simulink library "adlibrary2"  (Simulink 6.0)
settings: Solver=ode45  StartTime=0.0  StopTime=10.0  RelTol=1e-3
undefined symbols (not defined in the file or in its folder): adlibrary2, ADM, Bit, DDR, Generation, II, Location, Lower, SDRAM, SRAM, Width, XP, XPL, XRC, ZBT
libraries: xbsIndex_r3 x581, adlibrary2 x2
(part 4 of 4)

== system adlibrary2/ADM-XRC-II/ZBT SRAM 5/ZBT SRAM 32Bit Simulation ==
  d : Inport  Port=1  LatchInput=off
  a : Inport  Port=2  LatchInput=off
  w : Inport  Port=3  LatchInput=off
  r : Inport  Port=4  LatchInput=off
  be : Inport  Port=5  LatchInput=off
  Disregard Subsystem : xbsIndex_r3/Disregard Subsystem  Tag=discardX
  Gateway In6 : xbsIndex_r3/Gateway In  arith_type=Boolean  n_bits=1  bin_pt=0  quantization=Truncate  overflow=Wrap  period=1  timing_constraint=None  locs_specified=off  LOCs={}  needs_fixed_name=off  dbl_ovrd=on  show_param=off
  Gateway In7 : xbsIndex_r3/Gateway In  arith_type=Unsigned  n_bits=32  bin_pt=0  quantization=Truncate  overflow=Wrap  period=1  timing_constraint=None  locs_specified=off  LOCs={}  needs_fixed_name=off  dbl_ovrd=on  show_param=off
  Gateway Out{,1..4} (5 alike) : xbsIndex_r3/Gateway Out  hdl_port=off  timing_constraint=None  locs_specified=off  LOCs={}  needs_fixed_name=off  show_param=off
  S-Function : S-Function  FunctionName=zbt32
  q : Outport
  qv : Outport  Port=2
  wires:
  S-Function/2 -> Gateway In6/1
  Gateway In7/1 -> q/1
  Gateway In6/1 -> qv/1
  Gateway Out3/1 -> S-Function/4
  Gateway Out2/1 -> S-Function/3
  Gateway Out1/1 -> S-Function/2
  Gateway Out/1 -> S-Function/1
  S-Function/1 -> Gateway In7/1
  r/1 -> Gateway Out3/1
  w/1 -> Gateway Out2/1
  a/1 -> Gateway Out1/1
  d/1 -> Gateway Out/1
  Gateway Out4/1 -> S-Function/5
  be/1 -> Gateway Out4/1

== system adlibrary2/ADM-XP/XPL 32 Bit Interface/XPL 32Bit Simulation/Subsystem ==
  In1 : Inport  Port=1  LatchInput=off
  In2 : Inport  Port=2  LatchInput=off
  In9 : Inport  Port=3  LatchInput=off
  In3 : Inport  Port=4  LatchInput=off
  In4 : Inport  Port=5  LatchInput=off
  In5 : Inport  Port=6  LatchInput=off
  In6 : Inport  Port=7  LatchInput=off
  In7 : Inport  Port=8  LatchInput=off
  In8 : Inport  Port=9  LatchInput=off
  Disregard Subsystem : xbsIndex_r3/Disregard Subsystem  Tag=discardX
  Gateway In{,1,4..5} (4 alike) : xbsIndex_r3/Gateway In  arith_type=Boolean  n_bits=8  bin_pt=6  quantization=Truncate  overflow=Wrap  period=1  timing_constraint=None  locs_specified=off  LOCs={}  needs_fixed_name=off  dbl_ovrd=off  show_param=off
  Gateway In2 : xbsIndex_r3/Gateway In  arith_type=Unsigned  n_bits=32  bin_pt=0  quantization=Truncate  overflow=Wrap  period=1  timing_constraint=None  locs_specified=off  LOCs={}  needs_fixed_name=off  dbl_ovrd=off  show_param=off
  Gateway In3 : xbsIndex_r3/Gateway In  arith_type=Unsigned  n_bits=32  bin_pt=0  quantization=Truncate  overflow=Wrap  period=1  timing_constraint=None  locs_specified=off  LOCs={}  needs_fixed_name=off  dbl_ovrd=off  show_param=off
  Gateway In6 : xbsIndex_r3/Gateway In  arith_type=Unsigned  n_bits=16  bin_pt=0  quantization=Truncate  overflow=Wrap  period=1  timing_constraint=None  locs_specified=off  LOCs={}  needs_fixed_name=off  dbl_ovrd=off  show_param=off
  Gateway In7 : xbsIndex_r3/Gateway In  arith_type=Unsigned  n_bits=32  bin_pt=0  quantization=Truncate  overflow=Wrap  period=1  timing_constraint=None  locs_specified=off  LOCs={}  needs_fixed_name=off  dbl_ovrd=off  show_param=off
  Gateway In8 : xbsIndex_r3/Gateway In  arith_type=Unsigned  n_bits=4  bin_pt=0  quantization=Truncate  overflow=Wrap  period=1  timing_constraint=None  locs_specified=off  LOCs={}  needs_fixed_name=off  dbl_ovrd=off  show_param=off
  Out1 : Outport
  Out2 : Outport  Port=2
  Out9 : Outport  Port=3
  Out3 : Outport  Port=4
  Out4 : Outport  Port=5
  Out5 : Outport  Port=6
  Out6 : Outport  Port=7
  Out7 : Outport  Port=8
  Out8 : Outport  Port=9
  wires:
  In1/1 -> Gateway In7/1
  In2/1 -> Gateway In6/1
  In3/1 -> Gateway In5/1
  In4/1 -> Gateway In4/1
  In5/1 -> Gateway In3/1
  In6/1 -> Gateway In2/1
  In7/1 -> Gateway In1/1
  In8/1 -> Gateway In/1
  Gateway In/1 -> Out8/1
  Gateway In1/1 -> Out7/1
  Gateway In2/1 -> Out6/1
  Gateway In3/1 -> Out5/1
  Gateway In4/1 -> Out4/1
  Gateway In5/1 -> Out3/1
  Gateway In6/1 -> Out2/1
  Gateway In7/1 -> Out1/1
  In9/1 -> Gateway In8/1
  Gateway In8/1 -> Out9/1

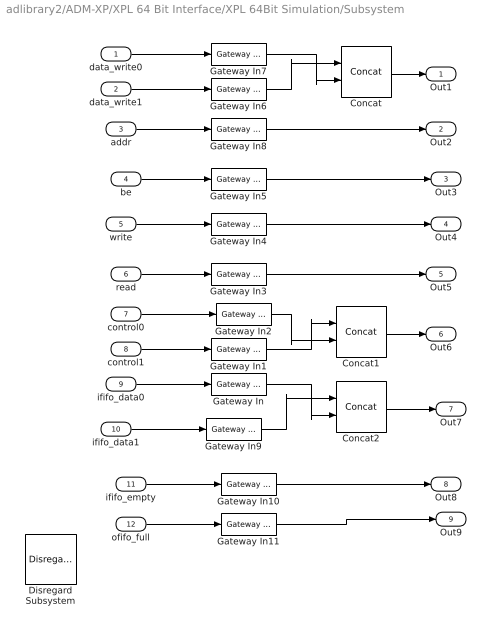
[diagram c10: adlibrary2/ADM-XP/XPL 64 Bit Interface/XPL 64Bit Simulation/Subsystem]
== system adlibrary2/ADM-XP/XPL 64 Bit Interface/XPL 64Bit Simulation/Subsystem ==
  data_write0 : Inport  Port=1  LatchInput=off
  data_write1 : Inport  Port=2  LatchInput=off
  addr : Inport  Port=3  LatchInput=off
  be : Inport  Port=4  LatchInput=off
  write : Inport  Port=5  LatchInput=off
  read : Inport  Port=6  LatchInput=off
  control0 : Inport  Port=7  LatchInput=off
  control1 : Inport  Port=8  LatchInput=off
  ififo_data0 : Inport  Port=9  LatchInput=off
  ififo_data1 : Inport  Port=10  LatchInput=off
  ififo_empty : Inport  Port=11  LatchInput=off
  ofifo_full : Inport  Port=12  LatchInput=off
  Concat : xbsIndex_r3/Concat  num_inputs=2  explicit_period=off  period=1  dbl_ovrd=off
  Concat1 : xbsIndex_r3/Concat  num_inputs=2  explicit_period=off  period=1  dbl_ovrd=off
  Concat2 : xbsIndex_r3/Concat  num_inputs=2  explicit_period=off  period=1  dbl_ovrd=off
  Disregard Subsystem : xbsIndex_r3/Disregard Subsystem  Tag=discardX
  Gateway In{,1..2,6..7,9} (6 alike) : xbsIndex_r3/Gateway In  arith_type=Unsigned  n_bits=32  bin_pt=0  quantization=Truncate  overflow=Wrap  period=1  timing_constraint=None  locs_specified=off  LOCs={}  needs_fixed_name=off  dbl_ovrd=off  show_param=off
  Gateway In10 : xbsIndex_r3/Gateway In  arith_type=Boolean  n_bits=8  bin_pt=6  quantization=Truncate  overflow=Wrap  period=1  timing_constraint=None  locs_specified=off  LOCs={}  needs_fixed_name=off  dbl_ovrd=off  show_param=off
  Gateway In11 : xbsIndex_r3/Gateway In  arith_type=Boolean  n_bits=8  bin_pt=6  quantization=Truncate  overflow=Wrap  period=1  timing_constraint=None  locs_specified=off  LOCs={}  needs_fixed_name=off  dbl_ovrd=off  show_param=off
  Gateway In3 : xbsIndex_r3/Gateway In  arith_type=Boolean  n_bits=32  bin_pt=0  quantization=Truncate  overflow=Wrap  period=1  timing_constraint=None  locs_specified=off  LOCs={}  needs_fixed_name=off  dbl_ovrd=off  show_param=off
  Gateway In4 : xbsIndex_r3/Gateway In  arith_type=Boolean  n_bits=8  bin_pt=6  quantization=Truncate  overflow=Wrap  period=1  timing_constraint=None  locs_specified=off  LOCs={}  needs_fixed_name=off  dbl_ovrd=off  show_param=off
  Gateway In5 : xbsIndex_r3/Gateway In  arith_type=Unsigned  n_bits=8  bin_pt=0  quantization=Truncate  overflow=Wrap  period=1  timing_constraint=None  locs_specified=off  LOCs={}  needs_fixed_name=off  dbl_ovrd=off  show_param=off
  Gateway In8 : xbsIndex_r3/Gateway In  arith_type=Unsigned  n_bits=16  bin_pt=0  quantization=Truncate  overflow=Wrap  period=1  timing_constraint=None  locs_specified=off  LOCs={}  needs_fixed_name=off  dbl_ovrd=off  show_param=off
  Out1 : Outport
  Out2 : Outport  Port=2
  Out3 : Outport  Port=3
  Out4 : Outport  Port=4
  Out5 : Outport  Port=5
  Out6 : Outport  Port=6
  Out7 : Outport  Port=7
  Out8 : Outport  Port=8
  Out9 : Outport  Port=9
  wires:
  Gateway In11/1 -> Out9/1
  Gateway In10/1 -> Out8/1
  Concat2/1 -> Out7/1
  Gateway In/1 -> Concat2/2
  Gateway In9/1 -> Concat2/1
  ofifo_full/1 -> Gateway In11/1
  ififo_empty/1 -> Gateway In10/1
  ififo_data1/1 -> Gateway In9/1
  Concat1/1 -> Out6/1
  Gateway In1/1 -> Concat1/1
  Gateway In2/1 -> Concat1/2
  Gateway In3/1 -> Out5/1
  Gateway In4/1 -> Out4/1
  Gateway In5/1 -> Out3/1
  Gateway In8/1 -> Out2/1
  Concat/1 -> Out1/1
  Gateway In7/1 -> Concat/2
  Gateway In6/1 -> Concat/1
  addr/1 -> Gateway In8/1
  ififo_data0/1 -> Gateway In/1
  control1/1 -> Gateway In1/1
  control0/1 -> Gateway In2/1
  read/1 -> Gateway In3/1
  write/1 -> Gateway In4/1
  be/1 -> Gateway In5/1
  data_write1/1 -> Gateway In6/1
  data_write0/1 -> Gateway In7/1

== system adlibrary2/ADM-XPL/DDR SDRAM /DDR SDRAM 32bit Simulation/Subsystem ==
  In1 : Inport  Port=1  LatchInput=off
  In2 : Inport  Port=2  LatchInput=off
  In3 : Inport  Port=3  LatchInput=off
  Disregard Subsystem : xbsIndex_r3/Disregard Subsystem  Tag=discardX
  g02 : xbsIndex_r3/Gateway In  arith_type=Unsigned  n_bits=3  bin_pt=0  quantization=Truncate  overflow=Wrap  period=1  timing_constraint=None  locs_specified=off  LOCs={}  needs_fixed_name=off  dbl_ovrd=off  show_param=off
  go0 : xbsIndex_r3/Gateway In  arith_type=Unsigned  n_bits=32  bin_pt=0  quantization=Truncate  overflow=Wrap  period=1  timing_constraint=None  locs_specified=off  LOCs={}  needs_fixed_name=off  dbl_ovrd=off  show_param=off
  go1 : xbsIndex_r3/Gateway In  arith_type=Boolean  n_bits=32  bin_pt=0  quantization=Truncate  overflow=Wrap  period=1  timing_constraint=None  locs_specified=off  LOCs={}  needs_fixed_name=off  dbl_ovrd=off  show_param=off
  Out1 : Outport
  Out2 : Outport  Port=2
  Out3 : Outport  Port=3
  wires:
  In1/1 -> go0/1
  In2/1 -> go1/1
  In3/1 -> g02/1
  go0/1 -> Out1/1
  go1/1 -> Out2/1
  g02/1 -> Out3/1

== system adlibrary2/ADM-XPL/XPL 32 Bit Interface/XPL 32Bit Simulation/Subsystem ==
  In1 : Inport  Port=1  LatchInput=off
  In2 : Inport  Port=2  LatchInput=off
  In9 : Inport  Port=3  LatchInput=off
  In3 : Inport  Port=4  LatchInput=off
  In4 : Inport  Port=5  LatchInput=off
  In5 : Inport  Port=6  LatchInput=off
  In6 : Inport  Port=7  LatchInput=off
  In7 : Inport  Port=8  LatchInput=off
  In8 : Inport  Port=9  LatchInput=off
  Disregard Subsystem : xbsIndex_r3/Disregard Subsystem  Tag=discardX
  Gateway In{,1,4..5} (4 alike) : xbsIndex_r3/Gateway In  arith_type=Boolean  n_bits=8  bin_pt=6  quantization=Truncate  overflow=Wrap  period=1  timing_constraint=None  locs_specified=off  LOCs={}  needs_fixed_name=off  dbl_ovrd=off  show_param=off
  Gateway In2 : xbsIndex_r3/Gateway In  arith_type=Unsigned  n_bits=32  bin_pt=0  quantization=Truncate  overflow=Wrap  period=1  timing_constraint=None  locs_specified=off  LOCs={}  needs_fixed_name=off  dbl_ovrd=off  show_param=off
  Gateway In3 : xbsIndex_r3/Gateway In  arith_type=Unsigned  n_bits=32  bin_pt=0  quantization=Truncate  overflow=Wrap  period=1  timing_constraint=None  locs_specified=off  LOCs={}  needs_fixed_name=off  dbl_ovrd=off  show_param=off
  Gateway In6 : xbsIndex_r3/Gateway In  arith_type=Unsigned  n_bits=16  bin_pt=0  quantization=Truncate  overflow=Wrap  period=1  timing_constraint=None  locs_specified=off  LOCs={}  needs_fixed_name=off  dbl_ovrd=off  show_param=off
  Gateway In7 : xbsIndex_r3/Gateway In  arith_type=Unsigned  n_bits=32  bin_pt=0  quantization=Truncate  overflow=Wrap  period=1  timing_constraint=None  locs_specified=off  LOCs={}  needs_fixed_name=off  dbl_ovrd=off  show_param=off
  Gateway In8 : xbsIndex_r3/Gateway In  arith_type=Unsigned  n_bits=4  bin_pt=0  quantization=Truncate  overflow=Wrap  period=1  timing_constraint=None  locs_specified=off  LOCs={}  needs_fixed_name=off  dbl_ovrd=off  show_param=off
  Out1 : Outport
  Out2 : Outport  Port=2
  Out9 : Outport  Port=3
  Out3 : Outport  Port=4
  Out4 : Outport  Port=5
  Out5 : Outport  Port=6
  Out6 : Outport  Port=7
  Out7 : Outport  Port=8
  Out8 : Outport  Port=9
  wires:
  Gateway In8/1 -> Out9/1
  In9/1 -> Gateway In8/1
  Gateway In7/1 -> Out1/1
  Gateway In6/1 -> Out2/1
  Gateway In5/1 -> Out3/1
  Gateway In4/1 -> Out4/1
  Gateway In3/1 -> Out5/1
  Gateway In2/1 -> Out6/1
  Gateway In1/1 -> Out7/1
  Gateway In/1 -> Out8/1
  In8/1 -> Gateway In/1
  In7/1 -> Gateway In1/1
  In6/1 -> Gateway In2/1
  In5/1 -> Gateway In3/1
  In4/1 -> Gateway In4/1
  In3/1 -> Gateway In5/1
  In2/1 -> Gateway In6/1
  In1/1 -> Gateway In7/1

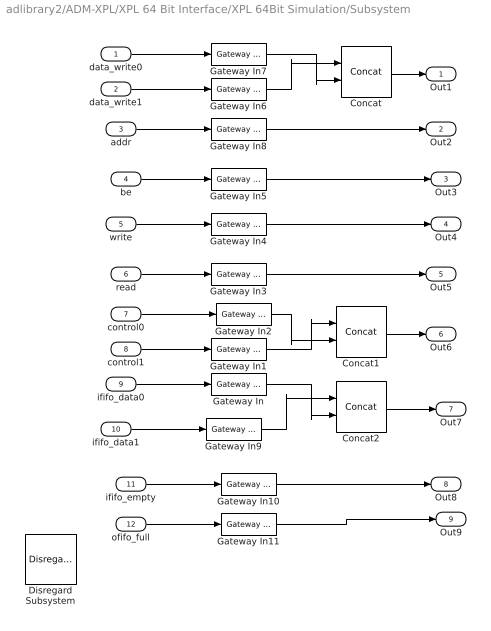
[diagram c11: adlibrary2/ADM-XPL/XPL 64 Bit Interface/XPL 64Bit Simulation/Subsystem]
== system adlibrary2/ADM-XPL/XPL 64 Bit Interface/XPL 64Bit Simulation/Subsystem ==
  data_write0 : Inport  Port=1  LatchInput=off
  data_write1 : Inport  Port=2  LatchInput=off
  addr : Inport  Port=3  LatchInput=off
  be : Inport  Port=4  LatchInput=off
  write : Inport  Port=5  LatchInput=off
  read : Inport  Port=6  LatchInput=off
  control0 : Inport  Port=7  LatchInput=off
  control1 : Inport  Port=8  LatchInput=off
  ififo_data0 : Inport  Port=9  LatchInput=off
  ififo_data1 : Inport  Port=10  LatchInput=off
  ififo_empty : Inport  Port=11  LatchInput=off
  ofifo_full : Inport  Port=12  LatchInput=off
  Concat : xbsIndex_r3/Concat  num_inputs=2  explicit_period=off  period=1  dbl_ovrd=off
  Concat1 : xbsIndex_r3/Concat  num_inputs=2  explicit_period=off  period=1  dbl_ovrd=off
  Concat2 : xbsIndex_r3/Concat  num_inputs=2  explicit_period=off  period=1  dbl_ovrd=off
  Disregard Subsystem : xbsIndex_r3/Disregard Subsystem  Tag=discardX
  Gateway In{,1..2,6..7,9} (6 alike) : xbsIndex_r3/Gateway In  arith_type=Unsigned  n_bits=32  bin_pt=0  quantization=Truncate  overflow=Wrap  period=1  timing_constraint=None  locs_specified=off  LOCs={}  needs_fixed_name=off  dbl_ovrd=off  show_param=off
  Gateway In10 : xbsIndex_r3/Gateway In  arith_type=Boolean  n_bits=8  bin_pt=6  quantization=Truncate  overflow=Wrap  period=1  timing_constraint=None  locs_specified=off  LOCs={}  needs_fixed_name=off  dbl_ovrd=off  show_param=off
  Gateway In11 : xbsIndex_r3/Gateway In  arith_type=Boolean  n_bits=8  bin_pt=6  quantization=Truncate  overflow=Wrap  period=1  timing_constraint=None  locs_specified=off  LOCs={}  needs_fixed_name=off  dbl_ovrd=off  show_param=off
  Gateway In3 : xbsIndex_r3/Gateway In  arith_type=Boolean  n_bits=32  bin_pt=0  quantization=Truncate  overflow=Wrap  period=1  timing_constraint=None  locs_specified=off  LOCs={}  needs_fixed_name=off  dbl_ovrd=off  show_param=off
  Gateway In4 : xbsIndex_r3/Gateway In  arith_type=Boolean  n_bits=8  bin_pt=6  quantization=Truncate  overflow=Wrap  period=1  timing_constraint=None  locs_specified=off  LOCs={}  needs_fixed_name=off  dbl_ovrd=off  show_param=off
  Gateway In5 : xbsIndex_r3/Gateway In  arith_type=Unsigned  n_bits=8  bin_pt=0  quantization=Truncate  overflow=Wrap  period=1  timing_constraint=None  locs_specified=off  LOCs={}  needs_fixed_name=off  dbl_ovrd=off  show_param=off
  Gateway In8 : xbsIndex_r3/Gateway In  arith_type=Unsigned  n_bits=16  bin_pt=0  quantization=Truncate  overflow=Wrap  period=1  timing_constraint=None  locs_specified=off  LOCs={}  needs_fixed_name=off  dbl_ovrd=off  show_param=off
  Out1 : Outport
  Out2 : Outport  Port=2
  Out3 : Outport  Port=3
  Out4 : Outport  Port=4
  Out5 : Outport  Port=5
  Out6 : Outport  Port=6
  Out7 : Outport  Port=7
  Out8 : Outport  Port=8
  Out9 : Outport  Port=9
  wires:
  data_write0/1 -> Gateway In7/1
  data_write1/1 -> Gateway In6/1
  be/1 -> Gateway In5/1
  write/1 -> Gateway In4/1
  read/1 -> Gateway In3/1
  control0/1 -> Gateway In2/1
  control1/1 -> Gateway In1/1
  ififo_data0/1 -> Gateway In/1
  addr/1 -> Gateway In8/1
  Gateway In6/1 -> Concat/1
  Gateway In7/1 -> Concat/2
  Concat/1 -> Out1/1
  Gateway In8/1 -> Out2/1
  Gateway In5/1 -> Out3/1
  Gateway In4/1 -> Out4/1
  Gateway In3/1 -> Out5/1
  Gateway In2/1 -> Concat1/2
  Gateway In1/1 -> Concat1/1
  Concat1/1 -> Out6/1
  ififo_data1/1 -> Gateway In9/1
  ififo_empty/1 -> Gateway In10/1
  ofifo_full/1 -> Gateway In11/1
  Gateway In9/1 -> Concat2/1
  Gateway In/1 -> Concat2/2
  Concat2/1 -> Out7/1
  Gateway In10/1 -> Out8/1
  Gateway In11/1 -> Out9/1

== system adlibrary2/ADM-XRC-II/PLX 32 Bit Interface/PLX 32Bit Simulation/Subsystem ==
  In1 : Inport  Port=1  LatchInput=off
  In2 : Inport  Port=2  LatchInput=off
  In9 : Inport  Port=3  LatchInput=off
  In3 : Inport  Port=4  LatchInput=off
  In4 : Inport  Port=5  LatchInput=off
  In5 : Inport  Port=6  LatchInput=off
  In6 : Inport  Port=7  LatchInput=off
  In7 : Inport  Port=8  LatchInput=off
  In8 : Inport  Port=9  LatchInput=off
  Disregard Subsystem : xbsIndex_r3/Disregard Subsystem  Tag=discardX
  Gateway In{,1,4..5} (4 alike) : xbsIndex_r3/Gateway In  arith_type=Boolean  n_bits=8  bin_pt=6  quantization=Truncate  overflow=Wrap  period=1  timing_constraint=None  locs_specified=off  LOCs={}  needs_fixed_name=off  dbl_ovrd=off  show_param=off
  Gateway In2 : xbsIndex_r3/Gateway In  arith_type=Unsigned  n_bits=32  bin_pt=0  quantization=Truncate  overflow=Wrap  period=1  timing_constraint=None  locs_specified=off  LOCs={}  needs_fixed_name=off  dbl_ovrd=off  show_param=off
  Gateway In3 : xbsIndex_r3/Gateway In  arith_type=Unsigned  n_bits=32  bin_pt=0  quantization=Truncate  overflow=Wrap  period=1  timing_constraint=None  locs_specified=off  LOCs={}  needs_fixed_name=off  dbl_ovrd=off  show_param=off
  Gateway In6 : xbsIndex_r3/Gateway In  arith_type=Unsigned  n_bits=16  bin_pt=0  quantization=Truncate  overflow=Wrap  period=1  timing_constraint=None  locs_specified=off  LOCs={}  needs_fixed_name=off  dbl_ovrd=off  show_param=off
  Gateway In7 : xbsIndex_r3/Gateway In  arith_type=Unsigned  n_bits=32  bin_pt=0  quantization=Truncate  overflow=Wrap  period=1  timing_constraint=None  locs_specified=off  LOCs={}  needs_fixed_name=off  dbl_ovrd=off  show_param=off
  Gateway In8 : xbsIndex_r3/Gateway In  arith_type=Unsigned  n_bits=4  bin_pt=0  quantization=Truncate  overflow=Wrap  period=1  timing_constraint=None  locs_specified=off  LOCs={}  needs_fixed_name=off  dbl_ovrd=off  show_param=off
  Out1 : Outport
  Out2 : Outport  Port=2
  Out9 : Outport  Port=3
  Out3 : Outport  Port=4
  Out4 : Outport  Port=5
  Out5 : Outport  Port=6
  Out6 : Outport  Port=7
  Out7 : Outport  Port=8
  Out8 : Outport  Port=9
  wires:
  Gateway In8/1 -> Out9/1
  In9/1 -> Gateway In8/1
  Gateway In7/1 -> Out1/1
  Gateway In6/1 -> Out2/1
  Gateway In5/1 -> Out3/1
  Gateway In4/1 -> Out4/1
  Gateway In3/1 -> Out5/1
  Gateway In2/1 -> Out6/1
  Gateway In1/1 -> Out7/1
  Gateway In/1 -> Out8/1
  In8/1 -> Gateway In/1
  In7/1 -> Gateway In1/1
  In6/1 -> Gateway In2/1
  In5/1 -> Gateway In3/1
  In4/1 -> Gateway In4/1
  In3/1 -> Gateway In5/1
  In2/1 -> Gateway In6/1
  In1/1 -> Gateway In7/1

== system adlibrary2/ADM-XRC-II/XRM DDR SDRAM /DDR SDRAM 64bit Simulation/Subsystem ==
  In1 : Inport  Port=1  LatchInput=off
  In2 : Inport  Port=2  LatchInput=off
  In3 : Inport  Port=3  LatchInput=off
  Disregard Subsystem : xbsIndex_r3/Disregard Subsystem  Tag=discardX
  g02 : xbsIndex_r3/Gateway In  arith_type=Unsigned  n_bits=3  bin_pt=0  quantization=Truncate  overflow=Wrap  period=1  timing_constraint=None  locs_specified=off  LOCs={}  needs_fixed_name=off  dbl_ovrd=off  show_param=off
  go0 : xbsIndex_r3/Gateway In  arith_type=Unsigned  n_bits=32  bin_pt=0  quantization=Truncate  overflow=Wrap  period=1  timing_constraint=None  locs_specified=off  LOCs={}  needs_fixed_name=off  dbl_ovrd=off  show_param=off
  go1 : xbsIndex_r3/Gateway In  arith_type=Boolean  n_bits=32  bin_pt=0  quantization=Truncate  overflow=Wrap  period=1  timing_constraint=None  locs_specified=off  LOCs={}  needs_fixed_name=off  dbl_ovrd=off  show_param=off
  Out1 : Outport
  Out2 : Outport  Port=2
  Out3 : Outport  Port=3
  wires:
  In1/1 -> go0/1
  In2/1 -> go1/1
  In3/1 -> g02/1
  go0/1 -> Out1/1
  go1/1 -> Out2/1
  g02/1 -> Out3/1
